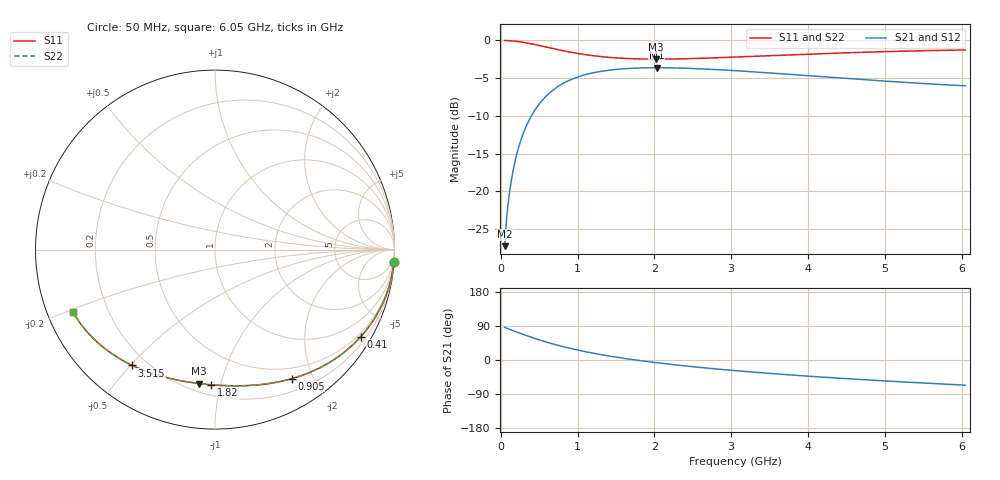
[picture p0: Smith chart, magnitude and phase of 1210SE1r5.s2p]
! AVX Thin Film Operation		Date: August 2001
! Description: Accu-P® Series, Thin Film, SMD, RF Capacitor
! Part Number: 12101J1R5ABT
! 50 MHz  -  6.05 GHz
! Serial Measurements
# mhz S db R 50
!	S11		S21		S12		S22
!	dB	Phase	dB	Phase	dB	Phase	dB	Phase
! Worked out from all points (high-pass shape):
!   401 points, 50 MHz to 6.05 GHz, reference 50 ohm
!   highest |S21| = -3.62 dB at 2.03 GHz (marker M1); lowest = -27.2 dB at 50 MHz (marker M2)
!   |S21| within 3 dB of the highest: 675.3 MHz to end of sweep
!   lowest |S11| = -2.5 dB at 2.015 GHz (marker M3), VSWR 7.05, Z = 12.5 - j42.9 ohm
!   |S11| at or under -10 dB: nowhere
!   |S22| runs from -2.5 to 0.0 dB; largest |S21 - S12| = 0
!   S11 on the Smith chart (normalised r, x): 50 MHz: 0, -29; 410 MHz: 0.39, -3.59; 905 MHz: 0.35, -1.70; 1.82 GHz: 0.27, -0.93; 3.515 GHz: 0.15, -0.51; 6.05 GHz: 0.08, -0.21
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50  -0.01 -3.9  -27.25 86.1  -27.25 86.1  -0.01 -3.9
65  -0.01 -5.1  -24.98 84.9  -24.98 84.9  -0.01 -5.1
125  -0.05 -9.8  -19.36 80.2  -19.36 80.2  -0.05 -9.8
185  -0.11 -14.5  -16.05 75.5  -16.05 75.5  -0.11 -14.5
230  -0.17 -17.9  -14.26 72.1  -14.26 72.1  -0.17 -17.9
290  -0.26 -22.3  -12.40 67.7  -12.40 67.7  -0.26 -22.3
410  -0.48 -30.8  -9.79 59.2  -9.79 59.2  -0.48 -30.8
515  -0.71 -37.8  -8.23 52.2  -8.23 52.2  -0.71 -37.8
635  -0.98 -45.1  -6.96 44.9  -6.96 44.9  -0.98 -45.1
905  -1.55 -59.3  -5.23 30.7  -5.23 30.7  -1.55 -59.3
1055  -1.81 -66.0  -4.67 24.0  -4.67 24.0  -1.81 -66.0
1415  -2.25 -79.6  -3.94 10.4  -3.94 10.4  -2.25 -79.6
1820  -2.46 -91.7  -3.65 -1.7  -3.65 -1.7  -2.46 -91.7
2015  -2.48 -96.7  -3.62 -6.8  -3.62 -6.8  -2.48 -96.7
2030  -2.48 -97.1  -3.62 -7.1  -3.62 -7.1  -2.48 -97.1
2060  -2.48 -97.8  -3.62 -7.8  -3.62 -7.8  -2.48 -97.8
2540  -2.39 -108.5  -3.74 -18.5  -3.74 -18.5  -2.39 -108.4
3050  -2.21 -118.0  -4.01 -28.0  -4.01 -28.0  -2.21 -118.0
3515  -2.01 -125.6  -4.32 -35.6  -4.32 -35.6  -2.01 -125.6
4055  -1.80 -133.4  -4.71 -43.4  -4.71 -43.4  -1.80 -133.3
5060  -1.47 -145.8  -5.43 -55.9  -5.43 -55.9  -1.47 -145.8
6050  -1.26 -156.5  -6.01 -66.5  -6.01 -66.5  -1.26 -156.5
